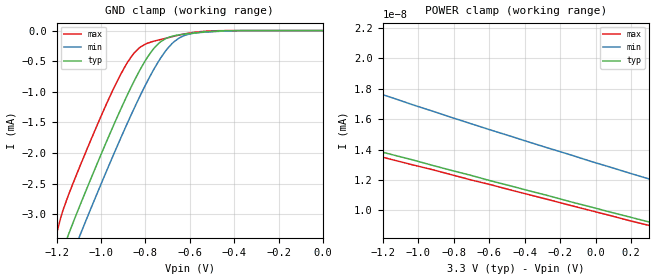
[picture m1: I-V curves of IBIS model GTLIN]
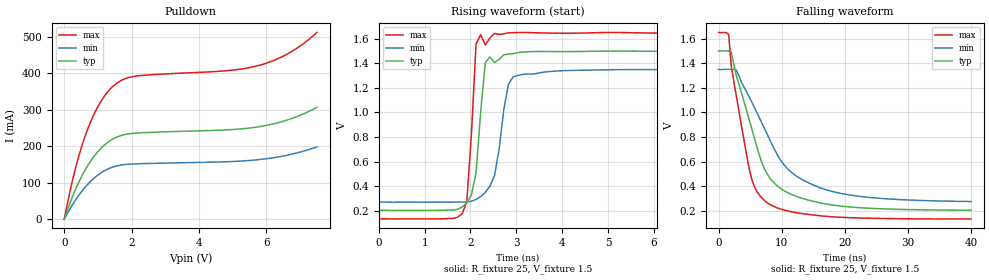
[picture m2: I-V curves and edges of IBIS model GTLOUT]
[IBIS Ver]   3.2
[Comment Char]   |_char
[File name]   gtl2034plus.ibs
[File Rev]   0
[Date]   May 2, 2006 5:03:45 PM
[Source]
[Notes]
[Disclaimer]
* Specialty Logic Products for Philips Semiconductors. Tempe, AZ
* K.Williams
*  Property of Philips Semiconductors *
*  Unauthorized reproduction and/or distribution is strictly *
*  prohibited.  (C) Copyright 2005 Philips Semiconductors. *
*  All rights reserved. *
*  PLEASE BE AWARE THAT IN THE ABSENCE OF A SIGNED, WRITTEN AGREEMENT *
*  TO THE CONTRARY, PHILIPS SEMICONDUCTORS (COMPANY) IS PROVIDING THE *
*  SPICE MODELS "AS IS" AND WITHOUT ANY WARRANTY, EXPRESSED OR IMPLIED.  *
*  Further, COMPANY assumes no liability for: 1) the accuracy of the *
*  SPICE models provided to your company; 2) the proper functioning of *
*  these SPICE models in your design or for any resulting applications;  *
*  or 3) infringement of patents, copyrights or intellectual property *
*  rights resulting from your use of these SPICE models. *
*  COMPANY provides SPICE models as a service to our customers.  You and *
*  your company shall not distribute, convey, sell or give these models  *
*  to anyone else without receiving prior written permission from *
*  COMPANY. *
*  COMPANY reserves the right to make changes to its products or to *
*  discontinue any semiconductor product or service without notice and *
*  advises its customers to obtain the latest version of relevant *
*  information to verify, before placing orders, that the information *
*  being relied on is current. *
*  Please be aware that your receipt and subsequent use of the SPICE *
*  information provided shall serve as acceptance of the terms and *
*  conditions of this agreement.  If you do not accept these terms, *
*  you should return the SPICE model and any other accompanying *
*  information immediately. *
[Copyright]
[Component]   GTL2034
Si_location Pin
Timing_location Pin
[Manufacturer]   Philips Semiconductor
[Package]
R_pkg   34.6m   28.0m   44.6m
L_pkg   2.04n   1.36n   2.32n
C_pkg   0.37pf   0.30pf   0.44pf
[Pin] signal_name   model_name
1   NC   NC
2   Bo0   GTLOUT
3   Bo1   GTLOUT
4   VREF   POWER
5   Bo2   GTLOUT
6   Bo3   GTLOUT
7   GND   GND
8   GND   GND
9   Bi3   GTLIN
10   Bi2   GTLIN
11   GND   GND
12   Bi1   GTLIN
13   Bi0   GTLIN
14   VCC   POWER
| Models and submodels in the file (2): GTLIN (Input), GTLOUT (Open_drain)
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[Model]   GTLIN
Model_type Input
Vinh=1.05
Vinl=0.95
C_comp   4.5p   4.5p   4.5p
[Model Spec]
[Temperature Range] 27   85   -40
[Voltage Range]   3.3   3.0   3.6
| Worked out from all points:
|   GND clamp passes 1 mA (typ) near -0.87 V on its own axis
|   POWER clamp passes 1 mA (typ) near -9.27 V on its own axis
[GND Clamp]
-1.5V     -1.188A    -662.4mA   -2.047A
-1.2V     -3.93mA    -4.411mA   -3.324mA
-1.14V    -3.272mA   -3.764mA   -2.627mA
-1.08V    -2.726mA   -3.214mA   -2.087mA
-920mV    -1.359mA   -1.832mA   -777.7uA
-860mV    -893.5uA   -1.346mA   -410.3uA
-820mV    -614.8uA   -1.039mA   -263.8uA
-730mV    -180.1uA   -442.6uA   -145.3uA
-680mV    -93.21uA   -213.4uA   -100.6uA
-620mV    -56.36uA   -75.67uA   -52.02uA
-420mV    -1.852uA   -4.796uA   -323.8nA
0V        0A         -3.307fA   0A
[POWER Clamp]
-10.7V    21.08A     19.98A     22.42A
-3.92V    22.57pA    30.75pA    21.66pA
-3.81V    22.2pA     30.1pA     21.34pA
-3.59V    21.46pA    28.82pA    20.69pA
-3.37V    20.72pA    27.57pA    19.98pA
-2.81V    18.93pA    24.67pA    18.33pA
-2.7V     18.53pA    24.13pA    18.02pA
-2.14V    16.77pA    21.5pA     16.33pA
-1.59V    15.05pA    19.16pA    14.68pA
-1.03V    13.32pA    16.94pA    12.99pA
-370mV    11.27pA    14.47pA    11.01pA
300mV     9.237pA    12.07pA    9.01pA
[Model]   GTLOUT
Model_type Open_drain
Vref=1.5
Vmeas=1.0
Rref=25
C_comp   5.5p   5.5p   5.5p
[Model Spec]
[Temperature Range] 27   85   -40
[Voltage Range]   3.3   3.0   3.6
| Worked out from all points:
|   slope of the pulldown table from 0 to 0.495 V, typ, clamps not added: 4.37 ohm
|   falling waveform, R_fixture 25, V_fixture 1.5: 20-80 % time 5.02ns typ, 7.37ns min, 3.29ns max; typ from 1.5 V to 0.204 V
|   rising waveform, R_fixture 25, V_fixture 1.5: 20-80 % time 186ps typ, 258ps min, 143ps max; typ from 0.202 V to 1.5 V
[Pulldown]
0V        -5.986uA   -6.235uA   -6.613uA
300mV     74.39mA    47.83mA    127.9mA
450mV     105.1mA    67.92mA    179.2mA
680mV     144.5mA    93.97mA    243.7mA
1.06V     191.7mA    125.1mA    319.4mA
1.29V     210.7mA    137.4mA    349.7mA
1.52V     223.5mA    145.1mA    370.6mA
2.12V     236mA      151.5mA    392.5mA
4.77V     244.7mA    157.2mA    407mA
5.76V     253.3mA    163.1mA    421.6mA
6.67V     273.5mA    176.5mA    455.8mA
7.5V      306.9mA    198.3mA    512.5mA
[Falling Waveform]
R_fixture=25
V_fixture=1.5
V_fixture_min=1.35
V_fixture_max=1.65
0s        1.5V       1.35V      1.65V
1.616ns   1.499V     1.35V      1.632V
2.02ns    1.49V      1.349V     1.376V
2.828ns   1.297V     1.343V     1.133V
4.848ns   942.2mV    1.127V     545.9mV
6.061ns   723.1mV    1.001V     358.2mV
7.677ns   502.2mV    825.4mV    266.8mV
10.91ns   348.5mV    543.2mV    199.3mV
16.57ns   259.5mV    379mV      157.2mV
40ns      204.1mV    275.2mV    132.8mV
[Rising Waveform]
R_fixture=25
V_fixture=1.5
V_fixture_min=1.35
V_fixture_max=1.65
0s        201.5mV    268.4mV    132mV
1.818ns   228.4mV    269.3mV    175.3mV
1.919ns   262.5mV    269.9mV    268.9mV
2.121ns   507.6mV    291mV      1.558V
2.222ns   1.005V     314mV      1.636V
2.323ns   1.407V     348mV      1.551V
2.525ns   1.407V     487.2mV    1.646V
2.828ns   1.477V     1.231V     1.65V
2.929ns   1.48V      1.291V     1.651V
10ns      1.5V       1.35V      1.65V
[Ramp]
R_load=25
dV/dt_r   7.791E-1/1.633E-10   7.194E-1/2.472E-10   8.284E-1/1.148E-10
dV/dt_f   7.775E-1/5.017E-9   7.144E-1/7.773E-9   8.280E-1/3.038E-9
|[End   GTLOUT
